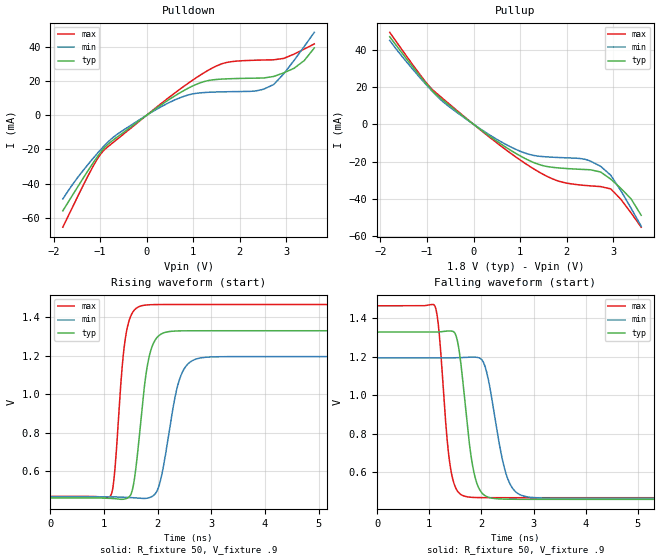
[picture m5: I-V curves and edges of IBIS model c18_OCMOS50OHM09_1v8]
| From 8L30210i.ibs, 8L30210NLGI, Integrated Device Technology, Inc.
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[Model] c18_OCMOS50OHM09_1v8
Model_type   Output
Polarity   Non-Inverting
|   typ   min   max
C_comp   2pF   1.5pF   2.5pF
Vmeas = .9
Rref = 50
Cref = 0
Vref = .9
|   typ   min   max
[Voltage range]   1.8V   1.650V   1.955V
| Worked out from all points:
|   slope of the pulldown table from 0 to 0.27 V, typ, clamps not added: 51.1 ohm
|   slope of the pullup table from 0 to 0.27 V, typ, clamps not added: 53.8 ohm
|   rising waveform, R_fixture 50, V_fixture .9: 20-80 % time 211ps typ, 279ps min, 166ps max; typ from 0.46 V to 1.33 V
|   falling waveform, R_fixture 50, V_fixture .9: 20-80 % time 221ps typ, 295ps min, 175ps max; typ from 1.33 V to 0.46 V
[Pulldown]
|Voltage   I (typ)   I (min)   I (max)
-1.8V     -55.9mA    -48.94mA   -65.46mA
-1.215V   -30.53mA   -27.32mA   -33.14mA
-939.7mV  -20.05mA   -18.68mA   -21.11mA
-160mV    -3.222mA   -2.741mA   -3.564mA
757.2mV   13.8mA     10.65mA    16.09mA
1.216V    19.56mA    13.24mA    24.58mA
1.629V    21.17mA    13.69mA    30.2mA
2.362V    21.71mA    14.34mA    32.2mA
2.728V    22.68mA    17.96mA    32.43mA
3.164V    27.45mA    32.03mA    35.75mA
3.382V    31.92mA    40.17mA    38.67mA
3.6V      39.34mA    48.5mA     41.74mA
[Pullup]
|Voltage   I (typ)   I (min)   I (max)
-1.8V     46.88mA    44.9mA     49.25mA
-1.169V   26.41mA    25.51mA    27.22mA
-893.8mV  18.25mA    17.86mA    18.85mA
-251.7mV  4.855mA    4.446mA    5.2mA
711.4mV   -12.58mA   -11.02mA   -13.94mA
1.216V    -19.65mA   -16.24mA   -22.69mA
1.72V     -23.12mA   -17.67mA   -29.47mA
2.362V    -24.2mA    -18.6mA    -32.68mA
2.728V    -25.54mA   -22.48mA   -33.37mA
2.946V    -29.38mA   -27.27mA   -34.6mA
3.382V    -39.91mA   -44.92mA   -47.42mA
3.6V      -48.73mA   -54.57mA   -55.1mA
[Ramp]
|   typ   min   max
dV/dt_r   0.525/0.212n   0.442/0.281n   0.601/0.166n
dV/dt_f   0.524/0.222n   0.44/0.296n   0.602/0.176n
R_load =   50.0000
[Rising Waveform]
R_fixture = 50
V_fixture = .9   |Vcc_typ
V_fixture_min = .825 |Vcc_min
V_fixture_max = .977 |Vcc_max
C_fixture = 0.0p
| Time   typ   min   max
0s        460.3mV    465.9mV    468.7mV
1.132ns   458mV      465.9mV    475.9mV
1.398ns   455.6mV    463.7mV    1.287V
1.541ns   515.1mV    461.7mV    1.427V
1.664ns   794.1mV    458.4mV    1.455V
1.797ns   1.128V     458.7mV    1.463V
1.94ns    1.274V     477mV      1.465V
2.396ns   1.328V     1.066V     1.465V
2.71ns    1.329V     1.181V     1.465V
9.49ns    1.329V     1.195V     1.465V
[Falling Waveform]
R_fixture = 50
V_fixture = .9   |Vcc_typ
V_fixture_min = .825 |Vcc_min
V_fixture_max = .977 |Vcc_max
C_fixture = 0.0p
| Time   typ   min   max
0s        1.329V     1.195V     1.465V
1.113ns   1.329V     1.194V     1.461V
1.398ns   1.334V     1.195V     640mV
1.531ns   1.293V     1.196V     507.3mV
1.655ns   1.045V     1.197V     478.7mV
1.807ns   675mV      1.199V     470.8mV
1.959ns   514.1mV    1.195V     469.2mV
2.472ns   461.1mV    593.1mV    468.7mV
2.786ns   460.4mV    479.3mV    468.7mV
9.49ns    460.3mV    465.9mV    468.7mV
